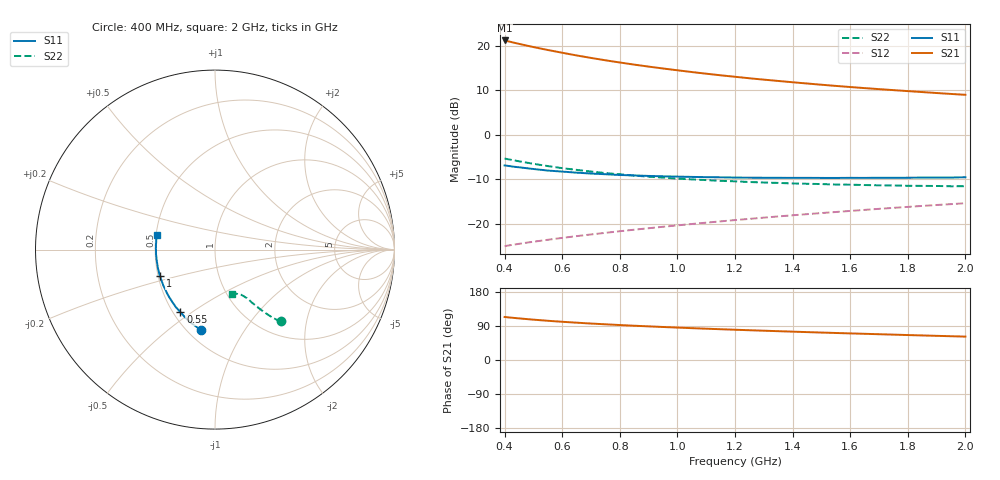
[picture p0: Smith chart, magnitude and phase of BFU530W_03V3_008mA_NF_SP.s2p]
! Filename:  P:\Prog\Test\Noise\ATS_data\Testdata_Net\06 Compressed Noise after Statistics\BFU530W_APM2013_09_A05_03p3V_008mA_NF_CM01_D.sf
! Date/Time: Tue 26/Mar/2013 18:06:07
! BFU530W_APM2013_09_A05_03p3V_1to25mA_NF_CM01_Bias5_R.sf
! Noise Parameter Data File
! BFU530W_APM2013_09_A05_03p3V_1to25mA_NF_CM01
! Date/time: Thu Mar 21 19:18:02 2013
! VAR V_out= 3.300000
! VAR I_out= 8.000000
! VAR V_in= 0.831600
! VAR I_in= 0.086010
! Device data file deembeded for feedlines and parallel
! Original file: \06 Compressed Noise after Statistics\BFU530W_APM2013_09_A05_03p3V_008mA_NF_CM01_R.sf
! Feed-files: PR019V01_070313_Feed1.s2p, PR019V01_070313_Feed2.s2p
! Parallel-file: PR019V01_070313_Par.s2p
# MHz S MA R 50
!  Freq-MHz  S11-mag  S11-arg  S21-mag  S21-arg  S12-mag  S12-arg  S22-mag  S22-arg
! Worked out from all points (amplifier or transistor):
!   37 points, 400 MHz to 2 GHz, reference 50 ohm
!   highest |S21| = 21.2 dB at 400 MHz (marker M1)
!   |S21| within 3 dB of that: start of sweep to 619.9 MHz
!   unconditionally stable (mu >= 1): 1.502 GHz to end of sweep
!   at 500 MHz: K = 0.67, MSG = 21.8 dB, |S12| = -24.0 dB
!   at 1.1 GHz: K = 0.94, MSG = 16.7 dB, |S12| = -19.7 dB
!   at 2 GHz: K = 1.02, MAG = 11.3 dB, |S12| = -15.3 dB
!   lowest NFmin = 0.69 dB at 440 MHz
!   S11 on the Smith chart (normalised r, x): 400 MHz: 0.58, -0.66; 550 MHz: 0.55, -0.45; 1 GHz: 0.51, -0.17; 2 GHz: 0.50, +0.09
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400  0.4546 -99.8  11.47 113.5  0.05639 57.3  0.5426 -47.5
420  0.445 -102.8  11.07 112.0  0.05786 57.1  0.5271 -48.3
433  0.4389 -104.6  10.82 111.0  0.05875 57.0  0.5173 -48.8
460  0.4289 -108.2  10.33 109.1  0.0606 56.9  0.4992 -49.6
500  0.4143 -113.4  9.674 106.5  0.06323 56.8  0.4737 -50.6
550  0.3979 -119.0  8.969 103.5  0.06651 57.1  0.4467 -51.7
600  0.3875 -124.3  8.35 100.8  0.06982 57.3  0.4235 -52.6
650  0.3767 -129.1  7.792 98.5  0.0731 57.5  0.4049 -53.3
700  0.3684 -133.6  7.307 96.2  0.07633 57.9  0.3881 -54.0
750  0.3619 -137.5  6.874 94.2  0.0796 58.3  0.3729 -54.5
800  0.3549 -141.4  6.491 92.3  0.08296 58.7  0.3614 -55.1
850  0.3507 -145.1  6.147 90.4  0.08628 59.0  0.3494 -55.5
950  0.3429 -151.4  5.561 87.1  0.09309 59.8  0.3315 -56.5
1000  0.3401 -154.4  5.308 85.5  0.09649 60.1  0.3228 -56.8
1100  0.3355 -159.8  4.862 82.6  0.1035 60.7  0.311 -57.9
1200  0.3321 -164.8  4.489 79.9  0.1106 61.1  0.3011 -58.8
1250  0.3309 -167.2  4.32 78.5  0.1142 61.3  0.2959 -59.3
1350  0.3297 -171.3  4.03 76.0  0.1216 61.6  0.2891 -60.4
1500  0.329 -177.4  3.656 72.4  0.1327 61.9  0.2806 -62.3
1650  0.3291 177.2  3.35 69.1  0.144 62.0  0.2736 -64.1
1750  0.3299 174.1  3.18 67.0  0.1517 61.9  0.2707 -65.5
2000  0.3347 166.3  2.817 61.7  0.1711 61.5  0.2652 -69.4
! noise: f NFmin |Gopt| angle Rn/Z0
400  0.6951  0.05116  110.1  0.0855
460  0.7137  0.06047  121  0.081
600  0.7191  0.04886  115.6  0.088
800  0.775  0.102  130  0.0786
1000  0.7832  0.118  139.9  0.0782
1200  0.8192  0.1468  149  0.0752
1400  0.8441  0.1696  157.8  0.072
1600  0.8637  0.1977  165.4  0.0666
1800  0.8752  0.2203  176.1  0.0679
2000  0.9235  0.2337  -175.8  0.0706
